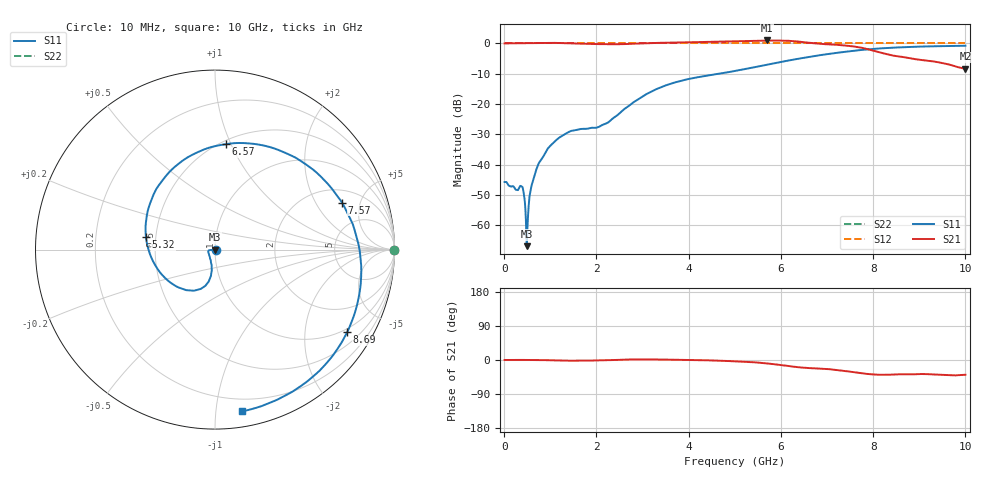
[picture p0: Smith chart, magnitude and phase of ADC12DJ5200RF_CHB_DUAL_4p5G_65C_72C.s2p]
! Texas Instruments, Inc.
! ADC12DJ5200RF - CH B S-Parameters (Dual Ch Mode, Fs = 4.5 GSPS, 65 degC case, 72 degC juntion)
! Port 1 represents the 100-ohm differenal input, Port 2 the digital output
! freq  dbS11  angS11  dbS21 angS21 dbS12 angS12 dbS22 angS22
# HZ S DB R 100
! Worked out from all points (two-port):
!   1000 points, 10 MHz to 10 GHz, reference 100 ohm
!   highest |S21| = 0.97 dB at 5.69 GHz (marker M1); lowest = -8.4 dB at 10 GHz (marker M2)
!   |S21| within 3 dB of the highest: start of sweep to 7.914 GHz
!   lowest |S11| = -66.8 dB at 490 MHz (marker M3), VSWR 1.00, Z = 100 + j0.0909 ohm
!   |S11| at or under -10 dB: start of sweep to 4.655 GHz
!   |S22| runs from 0.0 to 0.0 dB; largest |S21 - S12| = 0.74
!   S11 on the Smith chart (normalised r, x): 10 MHz: 1.01, -0.00; 5.32 GHz: 0.44, +0.07; 6.57 GHz: 0.53, +0.96; 7.57 GHz: 2.79, +3.39; 8.69 GHz: 0.87, -3.26; 10 GHz: 0.11, -1.18
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1e7  -45.69 -2.8  0.00 0.0  0.00 0.0  0.00 0.0
3.8e8  -47.17 -16.4  0.07 0.2  0.00 0.0  0.00 0.0
4.9e8  -66.84 93.5  0.09 0.2  0.00 0.0  0.00 0.0
5.2e8  -56.15 -177.4  0.10 0.1  0.00 0.0  0.00 0.0
5.8e8  -47.93 -158.5  0.11 0.1  0.00 0.0  0.00 0.0
6.5e8  -44.16 -162.0  0.12 0.0  0.00 0.0  0.00 0.0
9.2e8  -35.36 -172.3  0.19 -0.5  0.00 0.0  0.00 0.0
1.25e9  -30.53 -174.5  0.12 -1.5  0.00 0.0  0.00 0.0
1.68e9  -28.19 -167.0  -0.10 -1.7  0.00 0.0  0.00 0.0
2.22e9  -26.31 -127.8  -0.24 -0.7  0.00 0.0  0.00 0.0
3.34e9  -14.84 -101.2  0.17 1.4  0.00 0.0  0.00 0.0
4.23e9  -11.08 -126.9  0.44 -0.1  0.00 0.0  0.00 0.0
5.01e9  -9.07 -169.7  0.72 -3.5  0.00 0.0  0.00 0.0
5.32e9  -8.17 169.9  0.80 -5.2  0.00 0.0  0.00 0.0
5.69e9  -7.06 144.7  0.97 -9.0  0.00 0.0  0.00 0.0
6.57e9  -4.57 84.1  0.29 -20.8  0.00 0.0  0.00 0.0
6.67e9  -4.31 77.3  0.13 -21.8  0.00 0.0  0.00 0.0
7.09e9  -3.36 49.3  -0.33 -24.8  0.00 0.0  0.00 0.0
7.57e9  -2.45 20.4  -1.00 -31.9  0.00 0.0  0.00 0.0
8.34e9  -1.48 -18.1  -3.71 -38.9  0.00 0.0  0.00 0.0
8.69e9  -1.23 -32.1  -4.60 -37.8  0.00 0.0  0.00 0.0
1e10  -0.78 -80.5  -8.36 -39.0  0.00 0.0  0.00 0.0
